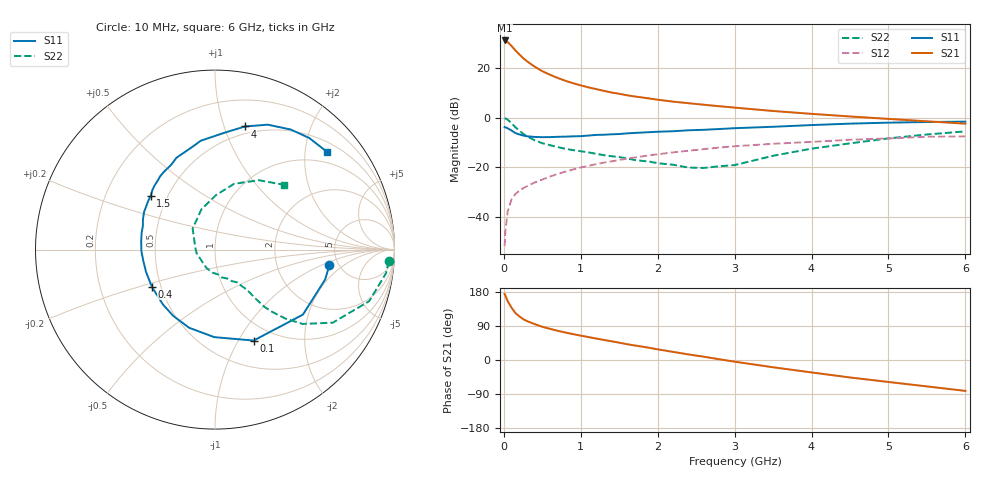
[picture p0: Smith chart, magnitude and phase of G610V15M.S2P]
! SIEMENS Small Signal Semiconductors
! BFG193
! Si NPN RF Bipolar Junction Transistor in SOT223
! VCE = 10 V  IC = 15 mA
! Common Emitter S-Parameters:  August  1996
# GHz  S  MA  R  50
!  f  S11  S21  S12  S22
! GHz  MAG  ANG  MAG  ANG  MAG  ANG  MAG  ANG
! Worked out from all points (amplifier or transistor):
!   36 points, 10 MHz to 6 GHz, reference 50 ohm
!   highest |S21| = 31.0 dB at 10 MHz (marker M1)
!   |S21| within 3 dB of that: start of sweep to 122.2 MHz
!   unconditionally stable (mu >= 1): 804.6 MHz to 2.584 GHz
!   at 250 MHz: K = 0.64, MSG = 26.2 dB, |S12| = -28.4 dB
!   at 1.4 GHz: K = 1.05, MAG = 12.4 dB, |S12| = -17.6 dB
!   at 6 GHz: K = 0.87, MSG = 2.5 dB, |S12| = -7.6 dB
!   S11 on the Smith chart (normalised r, x): 10 MHz: 4.23, -1.23; 100 MHz: 0.80, -1.16; 400 MHz: 0.45, -0.22; 1.5 GHz: 0.40, +0.31; 4 GHz: 0.43, +1.18; 6 GHz: 0.72, +2.49
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0.01  0.6435 -7.6  35.49 174.2  0.0026 86.0  0.9705 -3.8
0.02  0.6359 -15.2  35.21 170.0  0.0052 81.0  0.9617 -7.9
0.05  0.6092 -36.5  32.79 155.3  0.0129 73.8  0.9058 -18.5
0.1  0.5505 -67.0  27.53 138.1  0.0227 64.9  0.7725 -31.8
0.15  0.4877 -90.5  22.4 124.1  0.0291 57.9  0.6404 -40.3
0.2  0.4588 -108.3  18.67 115.3  0.0335 57.6  0.5488 -44.4
0.25  0.4364 -122.3  15.75 108.0  0.0379 55.8  0.4718 -47.4
0.3  0.4214 -133.6  13.56 102.7  0.0416 55.7  0.4225 -49.2
0.4  0.4082 -149.6  10.56 94.8  0.0493 56.1  0.3492 -50.5
0.5  0.4039 -162.2  8.563 87.6  0.0568 56.7  0.3052 -51.1
0.6  0.4048 -171.7  7.25 82.2  0.0652 56.8  0.2781 -52.0
0.7  0.4104 -179.2  6.265 77.1  0.0735 56.7  0.2556 -53.5
0.9  0.4192 167.3  4.907 68.3  0.0905 55.3  0.2214 -55.8
1.1  0.4351 157.3  4.047 60.5  0.1071 53.5  0.1992 -61.9
1.5  0.4669 140.1  3.003 45.7  0.1405 47.5  0.1606 -76.0
2.2  0.5311 117.5  2.09 21.4  0.1996 34.6  0.1127 -115.3
2.8  0.5884 101.9  1.691 2.0  0.2496 22.0  0.1048 -169.7
3.5  0.6531 85.4  1.356 -19.2  0.2972 5.8  0.1706 136.9
4  0.7062 76.3  1.188 -32.8  0.3242 -3.7  0.2371 108.6
4.5  0.7555 67.1  1.052 -46.1  0.3583 -13.8  0.3031 89.1
5.5  0.8138 49.9  0.841 -69.7  0.4109 -37.5  0.4572 57.7
6  0.8286 41.0  0.754 -81.5  0.4192 -51.2  0.5274 43.2
